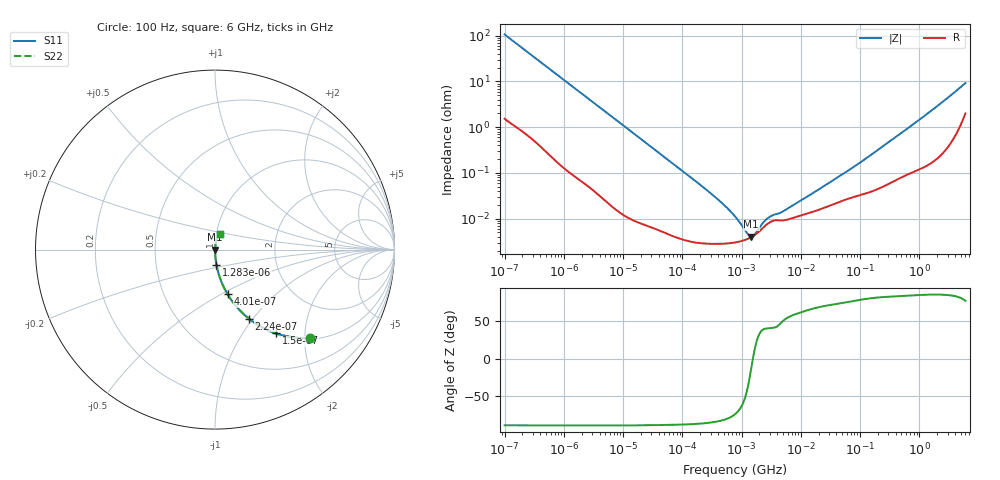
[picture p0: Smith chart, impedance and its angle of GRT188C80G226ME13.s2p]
!Murata Part Number: GRT188C80G226ME13
!These Parameters are Measured in Series Mode Connection
!Data Generated on Jun 19, 2026
!  o--ll--o
!Port1  Port2
!  o------o
!Operation Temp=25[degC], DC Bias Voltage=0[V]
!Freq. Start=100[Hz] Stop=6[GHz] 401[Steps]
# Hz S RI R 50
!Freq.(Hz) S11(Real) S11(Imag) S21(Real) S21(Imag) S12(Real) S12(Imag) S22(Real) S22(Imag)
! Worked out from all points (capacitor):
!   401 points, 100 Hz to 6 GHz, reference 50 ohm
!   read as one part in series: C = 14.9 uF near 109 Hz
!   lowest |Z| = 4.05 mohm at 1.45 MHz (marker M1)
!   series resonance near 1.553 MHz, so ESL is about 700 pH
!   S11 on the Smith chart (normalised r, x): 100 Hz: 1.03, -2.13; 150 Hz: 1.02, -1.43; 224 Hz: 1.01, -0.96; 401 Hz: 1.01, -0.54; 1.283 kHz: 1.00, -0.17; 6 GHz: 1.04, +0.18
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100  0.5305 -0.4919  0.4695 0.4919  0.4695 0.4919  0.5305 -0.4919
150  0.3396 -0.4663  0.6604 0.4663  0.6604 0.4663  0.3396 -0.4663
224  0.1902 -0.385  0.8098 0.385  0.8098 0.385  0.1902 -0.385
306  0.1134 -0.3098  0.8866 0.3098  0.8866 0.3098  0.1134 -0.3098
401  0.0707 -0.2493  0.9293 0.2493  0.9293 0.2493  0.0707 -0.2493
717  0.0241 -0.1473  0.9759 0.1473  0.9759 0.1473  0.0241 -0.1473
1283  0.0081 -0.084  0.9919 0.084  0.9919 0.084  0.0081 -0.084
2008  0.00359 -0.0541  0.9964 0.0541  0.9964 0.0541  0.00359 -0.0541
6433  0.000478 -0.0171  0.9995 0.0171  0.9995 0.0171  0.000478 -0.0171
40335  6.32e-05 -0.00276  0.9999 0.00276  0.9999 0.00276  6.32e-05 -0.00276
316350  2.83e-05 -0.00034  1 0.00034  1 0.00034  2.83e-05 -0.00034
517687  2.86e-05 -0.000192  1 0.000192  1 0.000192  2.86e-05 -0.000192
774597  3.03e-05 -0.000108  1 0.000108  1 0.000108  3.03e-05 -0.000108
926525  3.17e-05 -7.75e-05  1 7.75e-05  1 7.75e-05  3.17e-05 -7.75e-05
1449809  3.93e-05 -9.7e-06  1 9.7e-06  1 9.7e-06  3.93e-05 -9.7e-06
2713602  7.66e-05 6.56e-05  0.9999 -6.56e-05  0.9999 -6.56e-05  7.66e-05 6.56e-05
4856642  9.15e-05 0.000108  0.9999 -0.000108  0.9999 -0.000108  9.15e-05 0.000108
1.555665e7  0.00014 0.000326  0.9999 -0.000326  0.9999 -0.000326  0.00014 0.000326
7.797396e7  0.000299 0.00132  0.9997 -0.00132  0.9997 -0.00132  0.000299 0.00132
3.124326e8  0.000611 0.00481  0.9994 -0.00481  0.9994 -0.00481  0.000611 0.00481
1.873145e9  0.00263 0.0268  0.9974 -0.0268  0.9974 -0.0268  0.00263 0.0268
6e9  0.0271 0.0858  0.9729 -0.0858  0.9729 -0.0858  0.0271 0.0858
